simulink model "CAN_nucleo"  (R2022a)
settings: Solver=VariableStepAuto  StartTime=0.0  StopTime=10  RelTol=1e-3
undefined symbols (not defined in the file): bit, canChannel, Channel, identifier, Standard, Vector, VN1630A
libraries: slrealtimeutilitieslib x5, canmsglib x4, canlib x3

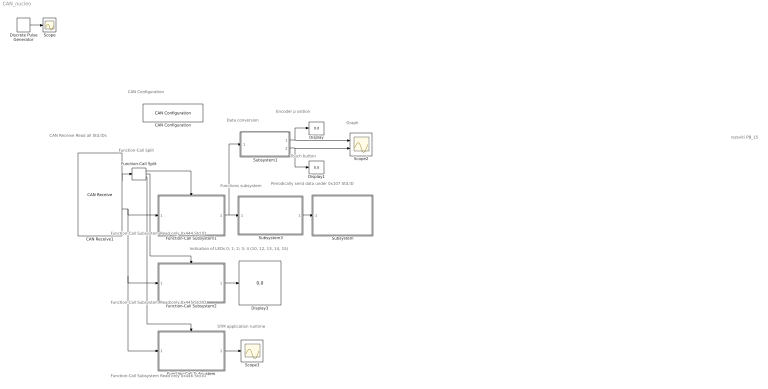
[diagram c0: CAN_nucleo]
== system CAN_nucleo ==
  note: Graph
  note: Encoder p osition
  note: Function-Call Split
  note: Function-Call Subsystem Read only 0x444 Std.ID
  note: CAN Configuration
  note: CAN Receive Read all Std.IDs
  note: Periodically send data under 0x107 Std.ID
  note: Functions subsystem
  note: Touch button
  note: rozsviti PB_15
  note: STM application runtime
  note: Indication of LEDs 0; 1; 2; 3; 4 (10, 12, 13, 14, 15)
  note: Function-Call Subsystem Read only 0x445 Std.ID
  note: Function-Call Subsystem Read only 0x446 Std.ID
  note: Data conversion
  CAN Configuration : canlib/CAN Configuration  BlockHandle=2.0002  Device=Vector VN1630A 1 (Channel 1)  DeviceMenu=Vector VN1630A 1 (Channel 1)  ObjConstructor=canChannel('Vector', 'VN1630A 1', 1)  BusSpeed=500000  EnableBitParameters=on  SJW=1  TSEG1=10  TSEG2=5  NSamples=1  AckMode=Normal
  CAN Receive1 : canlib/CAN Receive  BlockHandle=3.0002  Device=Vector VN1630A 1 (Channel 1)  DeviceMenu=Vector VN1630A 1 (Channel 1)  ObjConstructor=canChannel('Vector', 'VN1630A 1', 1)  EnableStandardIDsFilter=off  StdIDsCombo=Allow all  StandardIDs=0x444  EnableExtendedIDsFilter=off  ExtIDsCombo=Block all  ExtendedIDs=0  SampleTime=0.1  MsgsPerTimestep=all  InternalFilterUpdateStatus=on  BusOutput=off
  Discrete Pulse Generator : DiscretePulseGenerator  Period=10  PulseWidth=5
  Display : Display
  Display1 : Display
  Display3 : Display
  Function-Call Split : FunctionCallSplit  IconShape=distinctive  NumOutputPorts=3  OutputPortLayout=default
  Function-Call Subsystem : Subsystem  TreatAsAtomicUnit=on
  Function-Call Subsystem1 : Subsystem  TreatAsAtomicUnit=on
  Function-Call Subsystem2 : Subsystem  TreatAsAtomicUnit=on
  Scope : Scope
  Scope2 : Scope  NumInputPorts=2
  Scope3 : Scope
  Subsystem : Subsystem
  Subsystem1 : Subsystem
  Subsystem3 : Subsystem
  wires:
  Function-Call Subsystem/1(Out1) -> Scope3/1
  Discrete Pulse Generator/1 -> Scope/1
  CAN Receive1/2 -> Function-Call Subsystem1/1(In1), Function-Call Subsystem2/1(In1), Function-Call Subsystem/1(In1)
  Function-Call Subsystem2/1(Out1) -> Display3/1
  CAN Receive1/1 -> Function-Call Split/1
  Function-Call Split/1 -> Function-Call Subsystem1/Trigger
  Function-Call Split/2 -> Function-Call Subsystem2/Trigger
  Function-Call Split/3 -> Function-Call Subsystem/Trigger
  Subsystem3/1(Out1) -> Subsystem/1(In1)
  Function-Call Subsystem1/1(Out1) -> Subsystem1/1(In1), Subsystem3/1(In1)
  Subsystem1/1(Out1) -> Display/1, Scope2/1
  Subsystem1/2(Out2) -> Display1/1, Scope2/2

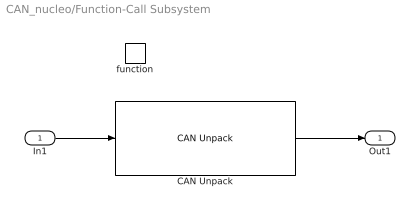
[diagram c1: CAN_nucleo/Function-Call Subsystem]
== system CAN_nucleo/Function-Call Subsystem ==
  In1 : Inport
  function : TriggerPort  TriggerType=function-call  VariantControl=(inherit)
  CAN Unpack : canmsglib/CAN Unpack  MsgList=(none)  MsgName=CAN Msg  MsgIDType=Standard (11-bit identifier)  MsgIdentifier=0x446  MsgLength=2  SignalInfo={}  IDPort=off  TimestampPort=off  ErrorPort=off  RemotePort=off  LengthPort=off  StatusPort=off  ApplyMinMax=off
  Out1 : Outport
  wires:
  In1/1 -> CAN Unpack/1
  CAN Unpack/1 -> Out1/1

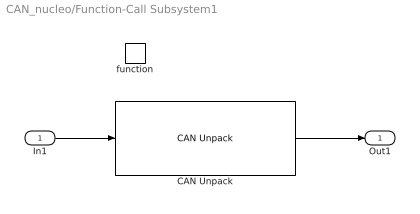
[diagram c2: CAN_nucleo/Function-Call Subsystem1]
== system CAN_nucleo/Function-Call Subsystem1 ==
  In1 : Inport
  function : TriggerPort  TriggerType=function-call  VariantControl=(inherit)
  CAN Unpack : canmsglib/CAN Unpack  MsgList=(none)  MsgName=CAN Msg  MsgIDType=Standard (11-bit identifier)  MsgIdentifier=0x444  MsgLength=2  SignalInfo={}  IDPort=off  TimestampPort=off  ErrorPort=off  RemotePort=off  LengthPort=off  StatusPort=off  ApplyMinMax=off
  Out1 : Outport
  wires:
  In1/1 -> CAN Unpack/1
  CAN Unpack/1 -> Out1/1

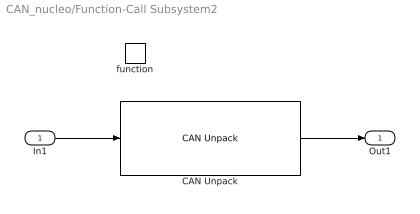
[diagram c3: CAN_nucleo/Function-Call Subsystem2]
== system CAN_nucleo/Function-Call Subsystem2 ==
  In1 : Inport
  function : TriggerPort  TriggerType=function-call  VariantControl=(inherit)
  CAN Unpack : canmsglib/CAN Unpack  MsgList=(none)  MsgName=CAN Msg  MsgIDType=Standard (11-bit identifier)  MsgIdentifier=0x445  MsgLength=5  SignalInfo={}  IDPort=off  TimestampPort=off  ErrorPort=off  RemotePort=off  LengthPort=off  StatusPort=off  ApplyMinMax=off
  Out1 : Outport
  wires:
  In1/1 -> CAN Unpack/1
  CAN Unpack/1 -> Out1/1

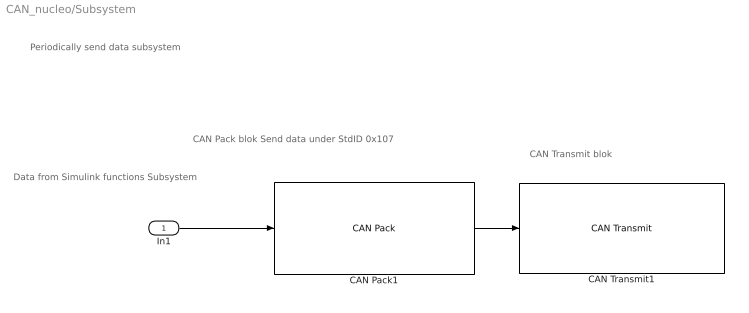
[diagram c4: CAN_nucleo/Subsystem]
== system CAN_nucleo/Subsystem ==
  note: CAN Pack blok Send data under StdID 0x107
  note: Data from Simulink functions Subsystem
  note: CAN Transmit blok
  note: Periodically send data subsystem
  In1 : Inport
  CAN Pack1 : canmsglib/CAN Pack  MsgList=(none)  MsgName=CAN Msg  MsgIDType=Standard (11-bit identifier)  MsgIdentifier=0x107  MsgLength=4  Remote=off  ApplyMinMax=off  BusOutput=off  SignalInfo={ 'Signal1', '0', '4', 'LE', 'unsigned', 'Standard', '0', '1', '0', '-Inf', 'Inf' }
  CAN Transmit1 : canlib/CAN Transmit  BlockHandle=217.0009  Device=Vector VN1630A 1 (Channel 1)  DeviceMenu=Vector VN1630A 1 (Channel 1)  ObjConstructor=canChannel('Vector', 'VN1630A 1', 1)  EnableEventTransmit=off  EnablePeriodicTransmit=on  MessagePeriod=0.100
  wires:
  CAN Pack1/1 -> CAN Transmit1/1
  In1/1 -> CAN Pack1/1

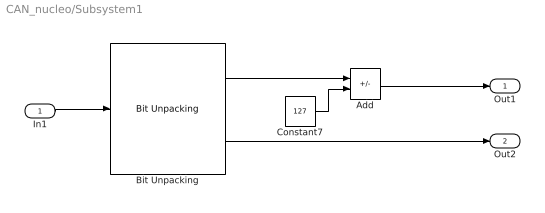
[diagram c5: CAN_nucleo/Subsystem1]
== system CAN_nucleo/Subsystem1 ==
  In1 : Inport
  Add : Sum  Inputs=+-
  Bit Unpacking : slrealtimeutilitieslib/Bit Unpacking  SignExtend=on
  Constant7 : Constant  Value=127
  Out1 : Outport
  Out2 : Outport  Port=2
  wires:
  Add/1 -> Out1/1
  Constant7/1 -> Add/2
  Bit Unpacking/1 -> Add/1
  In1/1 -> Bit Unpacking/1
  Bit Unpacking/2 -> Out2/1

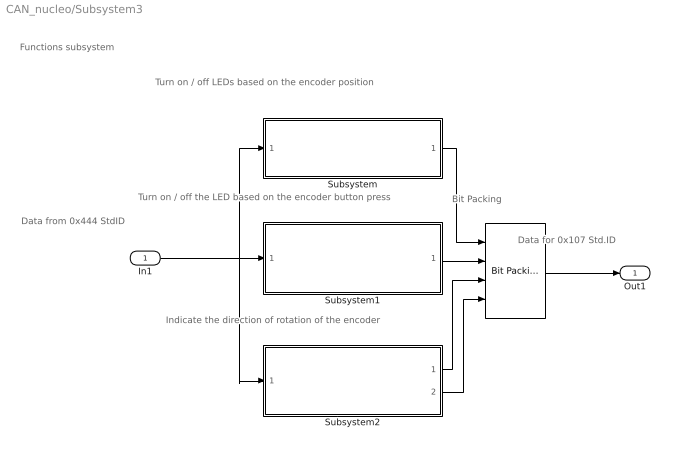
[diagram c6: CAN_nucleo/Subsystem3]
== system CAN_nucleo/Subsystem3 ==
  note: Bit Packing
  note: Data from 0x444 StdID
  note: Indicate the direction of rotation of the encoder
  note: Turn on / off LEDs based on the encoder position
  note: Turn on / off the LED based on the encoder button press
  note: Data for 0x107 Std.ID
  note: Functions subsystem
  In1 : Inport
  " " : slrealtimeutilitieslib/Bit Packing
  Subsystem : Subsystem
  Subsystem1 : Subsystem
  Subsystem2 : Subsystem
  Out1 : Outport
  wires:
  Subsystem2/2(Out2) -> " "/4
  In1/1 -> Subsystem/1(In1), Subsystem2/1(In1), Subsystem1/1(In1)
  Subsystem1/1(Out1) -> " "/2
  " "/1 -> Out1/1
  Subsystem2/1(Out1) -> " "/3
  Subsystem/1(Out1) -> " "/1

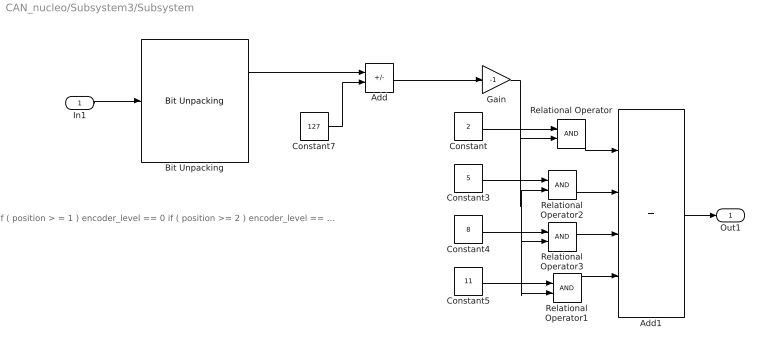
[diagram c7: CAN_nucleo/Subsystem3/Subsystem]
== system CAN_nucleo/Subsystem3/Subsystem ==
  note: if ( position > = 1 ) encoder_level == 0 if ( position >= 2 ) encoder_level == 1 if ( position > = 5 ) encoder_level == 2 if ( position > = 8 ) encoder_level == 3 if ( position > = 11 ) encoder_level == 4
  In1 : Inport
  Add : Sum  Inputs=+-
  Add1 : Sum  Inputs=++++
  Bit Unpacking : slrealtimeutilitieslib/Bit Unpacking  SignExtend=on
  Constant : Constant  Value=2
  Constant3 : Constant  Value=5
  Constant4 : Constant  Value=8
  Constant5 : Constant  Value=11
  Constant7 : Constant  Value=127
  Gain : Gain  Gain=-1
  Relational Operator{,1..3} (4 alike) : RelationalOperator  OutDataTypeStr=boolean  RndMeth=Simplest
  Out1 : Outport
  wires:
  Constant/1 -> Relational Operator/1
  Add/1 -> Gain/1
  Bit Unpacking/1 -> Add/1
  Relational Operator3/1 -> Add1/3
  Constant3/1 -> Relational Operator2/1
  Relational Operator/1 -> Add1/1
  Constant5/1 -> Relational Operator1/1
  Relational Operator1/1 -> Add1/4
  Relational Operator2/1 -> Add1/2
  Constant4/1 -> Relational Operator3/1
  Add1/1 -> Out1/1
  Constant7/1 -> Add/2
  In1/1 -> Bit Unpacking/1
  Gain/1 -> Relational Operator3/2, Relational Operator1/2, Relational Operator2/2, Relational Operator/2

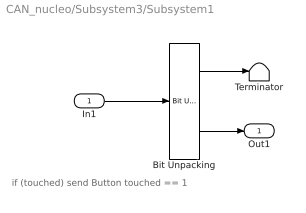
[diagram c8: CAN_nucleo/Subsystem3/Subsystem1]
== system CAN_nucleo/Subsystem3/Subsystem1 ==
  note: if (touched) send Button touched == 1
  In1 : Inport
  Bit Unpacking : slrealtimeutilitieslib/Bit Unpacking  SignExtend=on
  Terminator : Terminator
  Out1 : Outport
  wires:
  In1/1 -> Bit Unpacking/1
  Bit Unpacking/2 -> Out1/1
  Bit Unpacking/1 -> Terminator/1

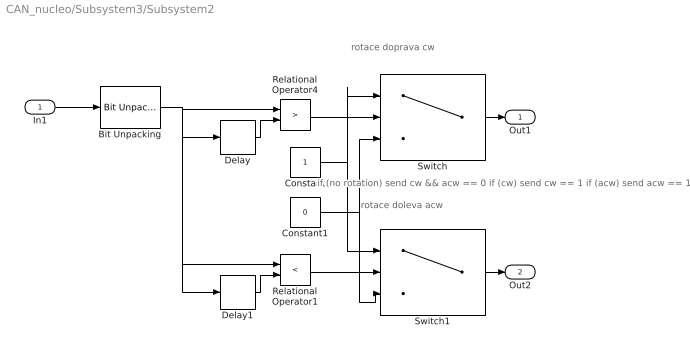
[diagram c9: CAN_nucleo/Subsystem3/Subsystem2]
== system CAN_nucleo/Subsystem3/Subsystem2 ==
  note: rotace doleva acw
  note: rotace doprava cw
  note: if (no rotation) send cw && acw == 0 if (cw) send cw == 1 if (acw) send acw == 1
  In1 : Inport
  Bit Unpacking : slrealtimeutilitieslib/Bit Unpacking  SignExtend=on
  Constant : Constant  OutDataTypeStr=uint8
  Constant1 : Constant  Value=0  OutDataTypeStr=uint8
  Delay : Delay  DelayLength=1  InitialCondition=0
  Delay1 : Delay  DelayLength=1  InitialCondition=0
  Relational Operator1 : RelationalOperator  Operator=<  OutDataTypeStr=boolean  RndMeth=Simplest
  Relational Operator4 : RelationalOperator  Operator=>  OutDataTypeStr=boolean  RndMeth=Simplest
  Switch : Switch  Criteria=u2 > Threshold  OutDataTypeStr=uint8
  Switch1 : Switch  Criteria=u2 > Threshold  OutDataTypeStr=uint8
  Out1 : Outport
  Out2 : Outport  Port=2
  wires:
  Relational Operator4/1 -> Switch/2
  Bit Unpacking/1 -> Delay1/1, Relational Operator1/1, Delay/1, Relational Operator4/1
  Delay/1 -> Relational Operator4/2
  In1/1 -> Bit Unpacking/1
  Constant/1 -> Switch/1, Switch1/1
  Constant1/1 -> Switch/3, Switch1/3
  Delay1/1 -> Relational Operator1/2
  Relational Operator1/1 -> Switch1/2
  Switch/1 -> Out1/1
  Switch1/1 -> Out2/1
